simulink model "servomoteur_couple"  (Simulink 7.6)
settings: Solver=ode14x  StartTime=0.0  StopTime=1  FixedStep=0.01  MaxStep=0.01  MinStep=0.001  RelTol=1e-3
InitFcn:
  | close all
StopFcn:
  | load servo_torque.mat
  | plot(x(1,:),x(2,:))
  | axis([0 0.02 0 0.1])
  | title('Couple (m.N)')
  | grid
libraries: fl_lib x8, nesl_utility x2, elec_lib x2

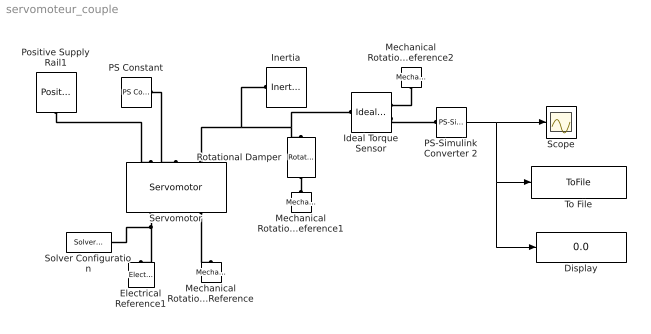
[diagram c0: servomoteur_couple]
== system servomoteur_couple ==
  Display : Display
  Electrical Reference1 : fl_lib/Electrical/Electrical Elements/Electrical Reference  DialogController=NetworkEngine.DynNeDlgSource  SystemSampleTime=-1  i_Log=off  LocalVarNames=|i  LocalVarDescs=|i  LocalVarLogging=[]
  Ideal Torque Sensor : fl_lib/Mechanical/Mechanical Sensors/Ideal Torque Sensor  DialogController=NetworkEngine.DynNeDlgSource  SystemSampleTime=-1  w_Log=off  t_Log=off  LocalVarNames=|w|t  LocalVarDescs=|w|t  LocalVarLogging=[0 0]
  Inertia : fl_lib/Mechanical/Rotational Elements/Inertia  DialogController=NetworkEngine.DynNeDlgSource  SystemSampleTime=-1  inertia=0.01 kg*m^2  initial_velocity=0 rad/s  t_Log=off  LocalVarNames=|t  LocalVarDescs=|t  LocalVarLogging=0
  Mechanical Rotational Reference : fl_lib/Mechanical/Rotational Elements/Mechanical Rotational Reference  DialogController=NetworkEngine.DynNeDlgSource  SystemSampleTime=-1  t_Log=off  LocalVarNames=|t  LocalVarDescs=|t  LocalVarLogging=[]
  Mechanical Rotational Reference1 : fl_lib/Mechanical/Rotational Elements/Mechanical Rotational Reference  DialogController=NetworkEngine.DynNeDlgSource  SystemSampleTime=-1  t_Log=off  LocalVarNames=|t  LocalVarDescs=|t  LocalVarLogging=0
  Mechanical Rotational Reference2 : fl_lib/Mechanical/Rotational Elements/Mechanical Rotational Reference  DialogController=NetworkEngine.DynNeDlgSource  SystemSampleTime=-1  t_Log=off  LocalVarNames=|t  LocalVarDescs=|t  LocalVarLogging=[]
  PS Constant : fl_lib/Physical Signals/Sources/PS Constant  DialogController=NetworkEngine.DynNeDlgSource  SystemSampleTime=-1  constant=5  LocalVarLogging=[]
  PS-Simulink Converter 2 : nesl_utility/PS-Simulink Converter  DialogController=NetworkEngine.DynNeUtilDlgSource  SystemSampleTime=-1  PhysicalDomain=network_engine_domain  LeftPortType=input  RightPortType=output  SubClassName=ps_output  Unit=N*m  AffineConversion=off
  Positive Supply Rail1 : elec_lib/Sources/Positive Supply Rail  DialogController=NetworkEngine.DynNeDlgSource  SystemSampleTime=-1  v0=12 V  current_Log=off  voltage_Log=off  power_Log=off  LocalVarNames=|current|voltage|power  LocalVarDescs=|Current (A)|Voltage (V)|Power (W)  LocalVarLogging=[0 0 0]
  Rotational Damper : fl_lib/Mechanical/Rotational Elements/Rotational Damper  DialogController=NetworkEngine.DynNeDlgSource  SystemSampleTime=-1  D=0.001 N*m/(rad/s)  t_Log=off  w_Log=off  LocalVarNames=|t|w  LocalVarDescs=|t|w  LocalVarLogging=[0 0]
  Scope : Scope
  Servomotor : elec_lib/Actuators & Drivers/Rotational Actuators/Servomotor  DialogController=NetworkEngine.DynNeDlgSource  SystemSampleTime=-1  w_t="[0  3.75e+03  7.5e+03  8e+03 ]"  T_t=[0.09 0.08 0.07 0 ]  Tc=0.02 s  eff=100  w_eff=3.75e+3 rpm  T_eff=0.08 N*m  Pbase=0 W  Res=3.5 Ohm  J=5e-06 kg*m^2  lam=1e-05 N*m/(rad/s)  speed0=0 rpm  LocalVarLogging=[]
  Solver Configuration : nesl_utility/Solver Configuration  DialogController=NetworkEngine.DynNeUtilDlgSource  SystemSampleTime=-1  PhysicalDomain=network_engine_domain  LeftPortType=input  RightPortType=generic  SubClassName=solver  Accelerate=off  Profile=off  ResidualTolerance=1e-1  MaxNonlinIter=12  MaxModeIter=2  DoFixedCost=off  UseLocalSampling=off  DoDC=off  LinearAlgebra=Sparse  LocalSolverSampleTime=.001  LocalSolverChoice=NE_BACKWARD_EULER_ADVANCER  UseLocalSolver=off
  To File : ToFile  Filename=servo_torque.mat  MatrixName=x
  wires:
  PS-Simulink Converter 2/1 -> Scope/1, To File/1, Display/1
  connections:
  Servomotor/LConn3 -- Ideal Torque Sensor/LConn1 -- Rotational Damper/LConn1 -- Inertia/LConn1
  Servomotor/RConn3 -- Mechanical Rotational Reference/LConn1
  Ideal Torque Sensor/RConn2 -- PS-Simulink Converter 2/LConn1
  PS Constant/RConn1 -- Servomotor/LConn2
  Positive Supply Rail1/RConn1 -- Servomotor/LConn1
  Servomotor/RConn1 -- Electrical Reference1/LConn1 -- Solver Configuration/RConn1
  Rotational Damper/RConn1 -- Mechanical Rotational Reference1/LConn1
  Mechanical Rotational Reference2/LConn1 -- Ideal Torque Sensor/RConn1
